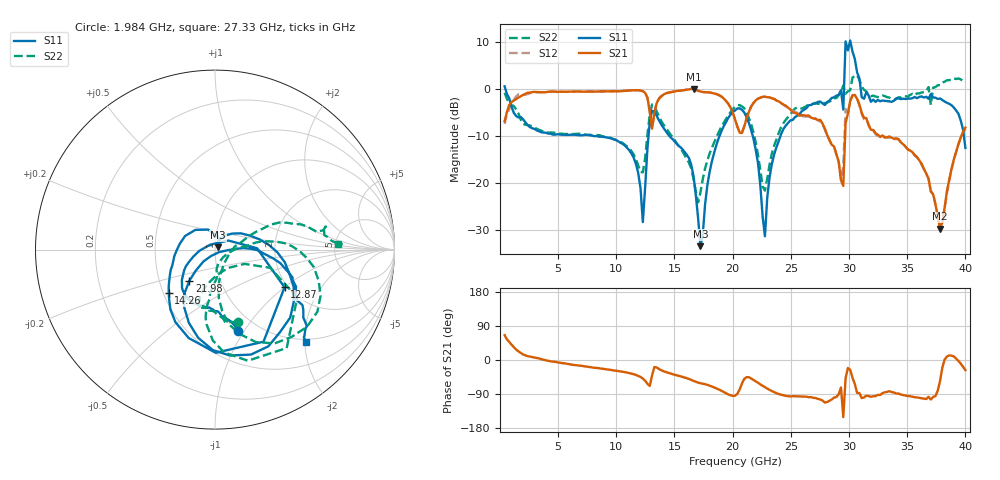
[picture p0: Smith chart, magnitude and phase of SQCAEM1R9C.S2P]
! Network Analyzer HP8722ES.07.66: Jul 25, 2000 Serial No. US39175408
! 26 Oct 2004  11:27:32
! Frequency  S11  S21  S12  S22
# HZ  S  DB R  50
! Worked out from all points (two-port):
!   201 points, 400 MHz to 40 GHz, reference 50 ohm
!   highest |S21| = -0.06 dB at 16.64 GHz (marker M1); lowest = -29.8 dB at 37.82 GHz (marker M2)
!   |S21| within 3 dB of the highest: 929.2 MHz to 12.75 GHz (11.82 GHz wide, 173 % of centre); 13.48 GHz to 19.57 GHz (6.096 GHz wide, 36.9 % of centre)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
!   lowest |S11| = -33.5 dB at 17.23 GHz (marker M3), VSWR 1.04, Z = 51.7 + j1.37 ohm
!   |S11| at or under -10 dB: 7.948 GHz to 12.77 GHz (4.822 GHz wide, 46.5 % of centre); 14.55 GHz to 18.88 GHz (4.333 GHz wide, 25.9 % of centre); 21.72 GHz to 24.12 GHz (2.396 GHz wide, 10.5 % of centre)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
!   |S22| runs from -24.1 to 2.9 dB; largest |S21 - S12| = 0.21
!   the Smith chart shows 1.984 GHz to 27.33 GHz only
!   S11 on the Smith chart (normalised r, x): 1.984 GHz: 0.80, -0.94; 12.87 GHz: 1.92, -1.00; 14.26 GHz: 0.53, -0.29; 21.98 GHz: 0.71, -0.26; 27.33 GHz: 0.94, -2.03
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4e8  0.49 -25.7  -6.90 65.6  -7.49 70.7  -0.88 -17.4
1.984e9  -6.51 -74.4  -1.34 14.6  -1.31 18.5  -7.46 -72.5
7.132e9  -9.90 -111.3  -0.65 -15.9  -0.68 -16.6  -9.72 -102.5
1.2874e10  -7.11 -28.5  -4.86 -68.5  -5.03 -69.4  -5.50 -30.4
1.3666e10  -6.73 -118.6  -2.13 -23.8  -2.09 -24.1  -5.91 -91.4
1.426e10  -9.05 -137.0  -1.00 -31.8  -1.02 -32.3  -8.37 -97.9
1.6636e10  -18.57 109.0  -0.06 -55.1  -0.06 -55.2  -19.18 -85.5
1.723e10  -33.47 38.6  -0.61 -61.4  -0.61 -61.6  -22.05 -12.2
2.02e10  -4.65 -51.7  -6.54 -94.3  -6.45 -94.4  -3.86 -23.5
2.1982e10  -13.00 -129.5  -2.50 -56.2  -2.53 -56.3  -11.41 -85.5
2.6932e10  -3.20 -44.0  -6.34 -99.8  -6.19 -100.2  -3.20 3.4
2.7328e10  -2.82 -45.5  -6.69 -102.6  -6.72 -102.2  -3.25 2.5
2.9506e10  -4.45 24.1  -20.66 -150.7  -16.34 -130.2  0.67 27.9
2.9704e10  10.04 -52.9  -7.36 -48.2  -4.31 -36.3  -1.09 -53.7
3.01e10  10.23 -70.2  -2.63 -25.8  -2.59 -27.0  -0.34 15.8
3.0496e10  6.32 -86.9  -1.33 -63.4  -1.43 -63.3  2.70 -15.5
3.0694e10  3.44 78.7  -2.17 -86.7  -2.08 -85.5  2.87 149.1
3.1288e10  -2.14 91.0  -6.21 -98.9  -6.50 -100.3  -0.25 139.8
3.1486e10  -0.74 -81.7  -6.28 -94.1  -6.43 -95.9  -0.59 -37.0
3.3466e10  -2.70 -63.0  -10.14 -82.4  -10.40 -82.7  -1.91 -23.1
3.7822e10  -2.09 -108.3  -29.75 -55.4  -29.21 -56.7  0.77 11.8
4e10  -12.61 -164.8  -8.28 -26.9  -8.50 -27.1  1.31 -20.7
